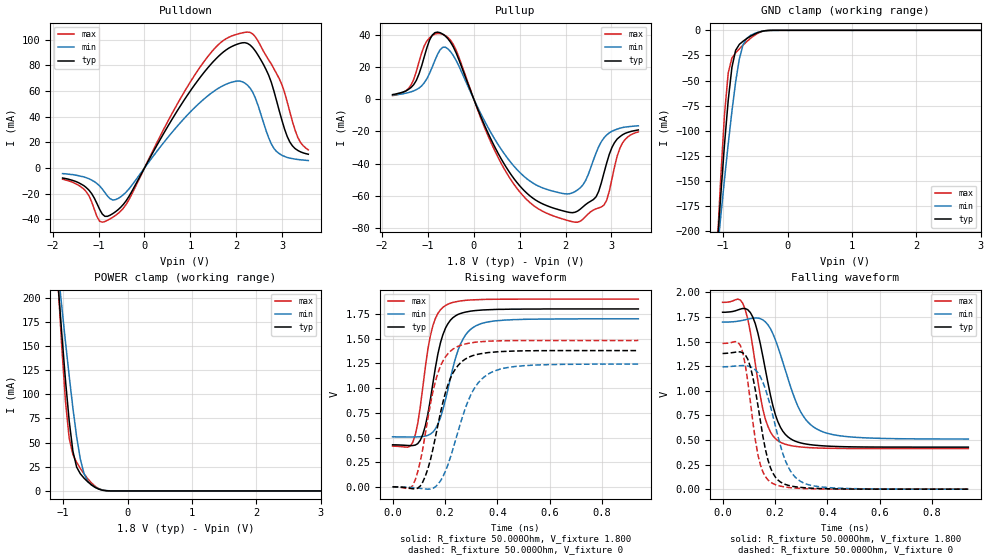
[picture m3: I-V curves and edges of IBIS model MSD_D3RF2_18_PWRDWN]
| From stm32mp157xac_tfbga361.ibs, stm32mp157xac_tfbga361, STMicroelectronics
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[Model] MSD_D3RF2_18_PWRDWN
Model_type   I/O
C_comp 2.550pF   2.465pF   2.675pF
Vinh = 1.150V
Vinl = 650.000mV
Vmeas = 900.000mV
Vref = 900.000mV
[Model Spec]
Vinh   1.150V   1.100V   1.200V
Vinl   650.000mV   600.000mV   700.000mV
Vmeas   900.000mV   850.000mV   950.000mV
Vref   900.000mV   850.000mV   950.000mV
[Temperature Range]   25.000   125.000   -40.000
[Voltage Range]   1.800V   1.700V   1.900V
[GND Clamp Reference]   0.00V   0.00V   0.00V
[Pulldown Reference]   0.00V   0.00V   0.00V
[POWER Clamp Reference]   1.800V   1.700V   1.900V
[Pullup Reference]   1.800V   1.700V   1.900V
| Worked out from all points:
|   slope of the pulldown table from 0 to 0.27 V, typ, clamps not added: 15.3 ohm
|   slope of the pullup table from 0 to 0.27 V, typ, clamps not added: 14.6 ohm
|   GND clamp passes 1 mA (typ) near -0.40 V on its own axis
|   POWER clamp passes 1 mA (typ) near -0.40 V on its own axis
|   rising waveform, R_fixture 50.000Ohm, V_fixture 1.800: 20-80 % time 58.7ps typ, 74.5ps min, 51.3ps max; typ from 0.426 V to 1.8 V
|   rising waveform, R_fixture 50.000Ohm, V_fixture 0: 20-80 % time 77ps typ, 97.3ps min, 68.9ps max; typ from 0.001 V to 1.38 V
|   falling waveform, R_fixture 50.000Ohm, V_fixture 1.800: 20-80 % time 68.9ps typ, 97.6ps min, 58.1ps max; typ from 1.8 V to 0.427 V
|   falling waveform, R_fixture 50.000Ohm, V_fixture 0: 20-80 % time 57.6ps typ, 80.3ps min, 48.6ps max; typ from 1.38 V to 0 V
[GND Clamp]
-1.785V   -904.7mA   -691.7mA   -1.214A
-1.094V   -216.3mA   -222.2mA   -217.4mA
-1.036V   -163.3mA   -184.8mA   -145.2mA
-978.8mV  -113.5mA   -148.4mA   -83.76mA
-921.2mV  -69.69mA   -113.3mA   -42.51mA
-863.6mV  -36.79mA   -80.49mA   -27.53mA
-806.1mV  -19.91mA   -51.37mA   -22.45mA
-748.5mV  -14mA      -28.45mA   -18.47mA
-690.9mV  -10.87mA   -14.34mA   -14.73mA
-575.8mV  -5.929mA   -5.08mA    -8.007mA
-287.9mV  -82.85uA   -135.6uA   -69.2uA
3.57V     41.7nA     685.7nA    4.362nA
[Power Clamp]
-1.77V    886.2mA    693mA      1.163A
-1.079V   214.1mA    227.9mA    214.3mA
-1.021V   162.4mA    190.6mA    148.6mA
-963.6mV  114.3mA    154.1mA    92.64mA
-906.1mV  72.38mA    118.8mA    54.46mA
-848.5mV  41.09mA    85.68mA    37.53mA
-790.9mV  24.71mA    56.22mA    29.66mA
-733.3mV  17.76mA    32.9mA     23.31mA
-618.2mV  9.462mA    10.19mA    12.58mA
-503mV    3.682mA    3.772mA    4.784mA
-272.7mV  36.6uA     118.7uA    36.53uA
3.585V    -62.58nA   -1.1uA     -6.985nA
[Pulldown]
-1.785V   -7.8mA     -4.4mA     -8.7mA
-1.267V   -15.3mA    -7.6mA     -18.6mA
-978.8mV  -32.1mA    -13.9mA    -41.44mA
-575.8mV  -32.49mA   -23.76mA   -35.4mA
1.209V    70.38mA    50.93mA    78.44mA
1.67V     88.85mA    63.32mA    97.95mA
2.188V    97.58mA    66.1mA     105.7mA
2.476V    87.76mA    48.51mA    98.76mA
2.821V    59.8mA     15.2mA     77.17mA
3.167V    20.2mA     7.7mA      43.7mA
3.339V    13.7mA     6.6mA      23.9mA
3.57V     10.7mA     5.8mA      14.1mA
[Pullup]
-1.77V    2.8mA      2.474mA    2.179mA
-1.367V   7.2mA      4.542mA    8.789mA
-1.136V   20.6mA     8.205mA    28.66mA
-906.1mV  39.62mA    19.85mA    39.36mA
-618.2mV  38.98mA    32.14mA    39.33mA
878.8mV   -49.38mA   -41.65mA   -52.89mA
1.455V    -64.25mA   -54.44mA   -68.75mA
2.203V    -70.07mA   -57.29mA   -76.21mA
2.664V    -60.5mA    -33.33mA   -67.93mA
2.836V    -45.7mA    -23.98mA   -65.62mA
3.182V    -23.3mA    -18.03mA   -30.45mA
3.585V    -19.1mA    -16.53mA   -20.3mA
[Ramp]
R_load=50.000Ohm
dV/dt_r   825.630mV/68.500ps  729.899mV/86.500ps  890.610mV/60.500ps
dV/dt_f   825.630mV/63.500ps  729.899mV/89.500ps  890.610mV/54.000ps
[Rising waveform]
R_fixture=50.000Ohm
V_fixture=1.800
V_fixture_min=1.700
V_fixture_max=1.900
0s        426.2mV    506.9mV    412.6mV
68ps      418.2mV    505.1mV    414mV
87ps      423.8mV    505.7mV    529.9mV
106ps     473.4mV    508.2mV    813.9mV
144ps     879.8mV    533.8mV    1.526V
173ps     1.345V     634.6mV    1.755V
202ps     1.606V     882.6mV    1.835V
259ps     1.754V     1.444V     1.881V
326ps     1.786V     1.639V     1.894V
938ps     1.8V       1.7V       1.9V
[Rising waveform]
R_fixture=50.000Ohm
V_fixture=0
0s        1.105mV    1mV        1.007mV
77ps      -18.48mV   -6.217mV   14.79mV
115ps     48.79mV    -17.57mV   381.8mV
144ps     269.5mV    -20.99mV   830.5mV
173ps     626.6mV    26.05mV    1.153V
202ps     955.2mV    161.3mV    1.316V
240ps     1.193V     470.3mV    1.409V
307ps     1.329V     974mV      1.46V
384ps     1.363V     1.167V     1.476V
938ps     1.379V     1.242V     1.482V
[Falling waveform]
R_fixture=50.000Ohm
V_fixture=1.800
V_fixture_min=1.700
V_fixture_max=1.900
0s        1.798V     1.698V     1.899V
77ps      1.836V     1.716V     1.889V
96ps      1.824V     1.728V     1.731V
115ps     1.751V     1.737V     1.45V
163ps     1.221V     1.701V     715.2mV
192ps     848.2mV    1.58V      542.9mV
221ps     628.4mV    1.367V     476.9mV
298ps     470.2mV    786.7mV    428.8mV
374ps     442mV      592.2mV    417.3mV
938ps     427.1mV    509.6mV    412.8mV
[Falling waveform]
R_fixture=50.000Ohm
V_fixture=0
0s        1.379V     1.243V     1.481V
68ps      1.395V     1.255V     1.46V
96ps      1.322V     1.252V     1.1V
125ps     1.009V     1.213V     501.8mV
144ps     698.6mV    1.143V     250.2mV
163ps     409.9mV    1.022V     128.9mV
192ps     163.3mV    746.1mV    56.96mV
250ps     39.42mV    227.7mV    17.79mV
317ps     13.63mV    54.87mV    5.427mV
938ps     -1.229uV   55.35uV    -5.719uV
